ORGANIZATION_BLOCK "OB1"
TITLE = "Main Program Sweep (Cycle)"
AUTHOR : CBARILE
VERSION : 0.1


VAR_TEMP
  OB1_EV_CLASS : BYTE ;	//Bits 0-3 = 1 (Coming event), Bits 4-7 = 1 (Event class 1)
  OB1_SCAN_1 : BYTE ;	//1 (Cold restart scan 1 of OB 1), 3 (Scan 2-n of OB 1)
  OB1_PRIORITY : BYTE ;	//1 (Priority of 1 is lowest)
  OB1_OB_NUMBR : BYTE ;	//1 (Organization block 1, OB1)
  OB1_RESERVED_1 : BYTE ;	//Reserved for system
  OB1_RESERVED_2 : BYTE ;	//Reserved for system
  OB1_PREV_CYCLE : INT ;	//Cycle time of previous OB1 scan (milliseconds)
  OB1_MIN_CYCLE : INT ;	//Minimum cycle time of OB1 (milliseconds)
  OB1_MAX_CYCLE : INT ;	//Maximum cycle time of OB1 (milliseconds)
  OB1_DATE_TIME : DATE_AND_TIME ;	//Date and time OB1 started
END_VAR
BEGIN
NETWORK
TITLE =LETTURA DATA E ORA
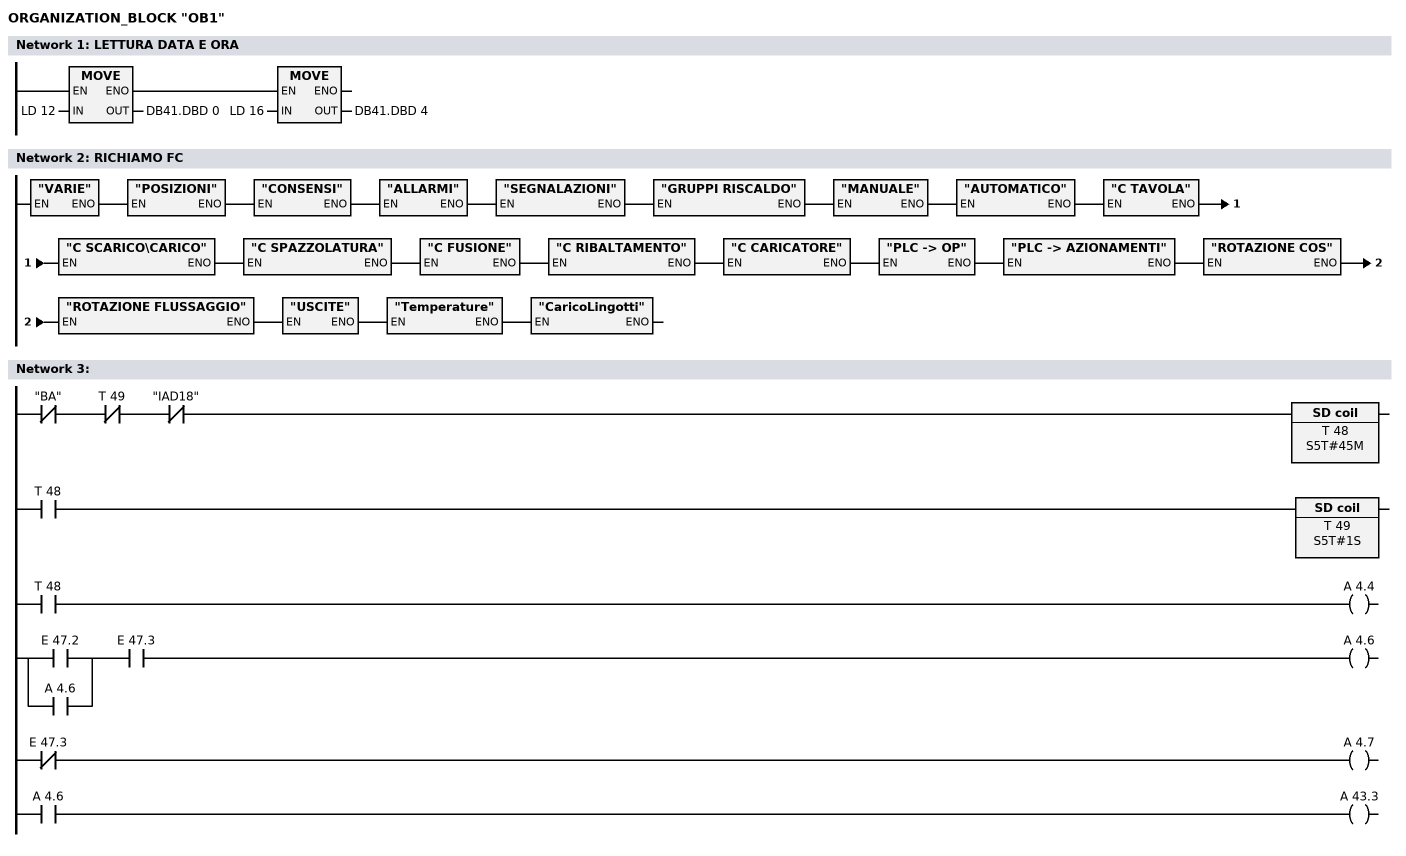
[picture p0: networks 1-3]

      L     LD    12;
      T     DB41.DBD    0;

      L     LD    16;
      T     DB41.DBD    4;
NETWORK
TITLE =RICHIAMO FC

      CALL "VARIE" ;
      CALL "POSIZIONI" ;
      CALL "CONSENSI" ;
      CALL "ALLARMI" ;
      CALL "SEGNALAZIONI" ;
      CALL "GRUPPI RISCALDO" ;
      CALL "MANUALE" ;
      CALL "AUTOMATICO" ;
      CALL "C TAVOLA" ;
      CALL "C SCARICO\CARICO" ;
      CALL "C SPAZZOLATURA" ;
      CALL "C FUSIONE" ;
      CALL "C RIBALTAMENTO" ;
      CALL "C CARICATORE" ;
      CALL "PLC -> OP" ;
      CALL "PLC -> AZIONAMENTI" ;
      CALL "ROTAZIONE COS" ;
      CALL "ROTAZIONE FLUSSAGGIO" ;
      CALL "USCITE" ;
      CALL "Temperature" ;
      CALL "CaricoLingotti" ;
NETWORK
TITLE =

      UN    "BA";
      UN    T     49;
      UN    "IAD18";
      L     S5T#45M;
      SE    T     48;
      U     T     48;
      L     S5T#1S;
      SE    T     49;
      U     T     48;
      =     A      4.4;
      U     E     47.2;
      O     A      4.6;
      U     E     47.3;
      =     A      4.6;
      UN    E     47.3;
      =     A      4.7;
      U     A      4.6;
      =     A     43.3;
END_ORGANIZATION_BLOCK

